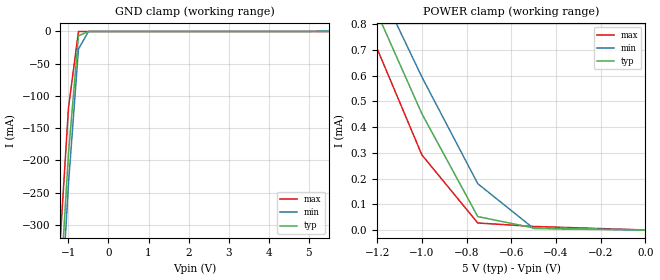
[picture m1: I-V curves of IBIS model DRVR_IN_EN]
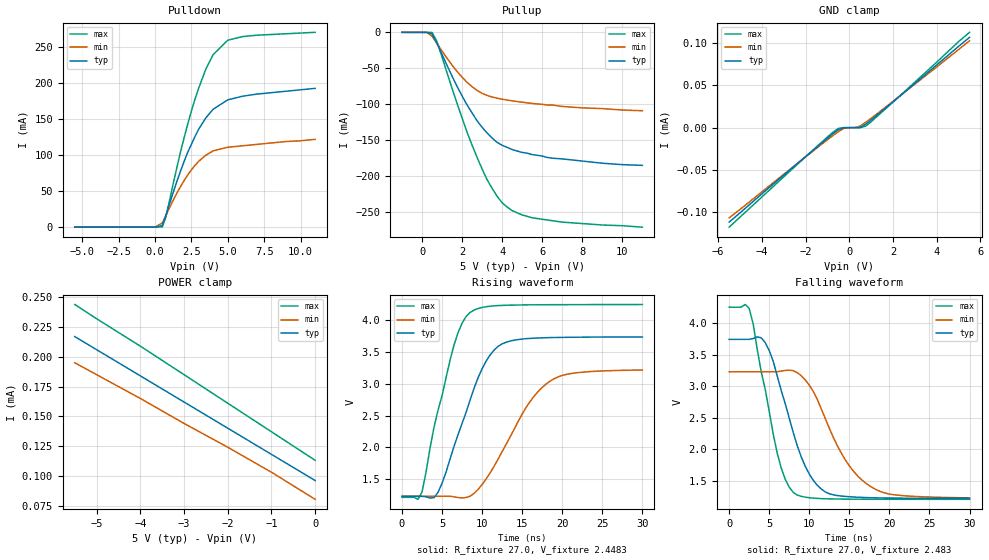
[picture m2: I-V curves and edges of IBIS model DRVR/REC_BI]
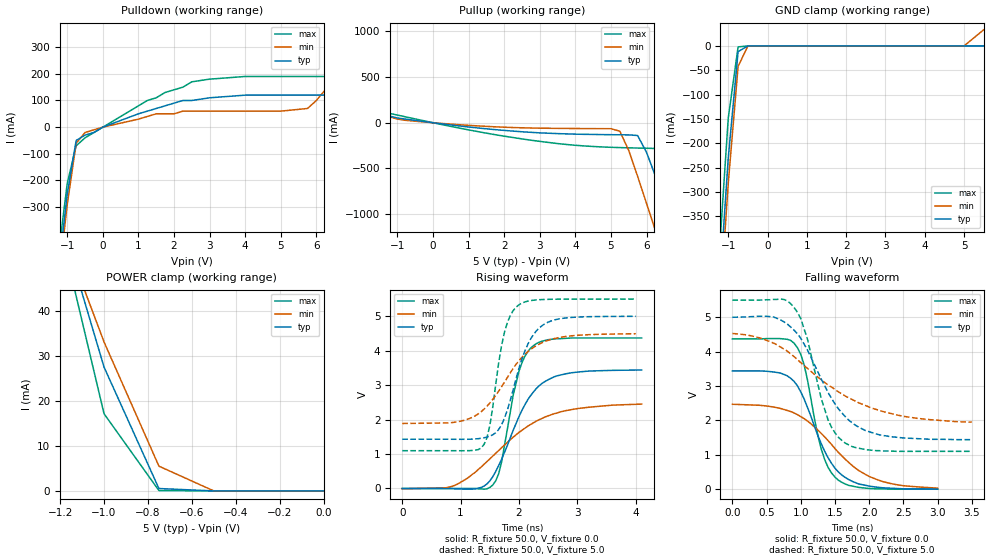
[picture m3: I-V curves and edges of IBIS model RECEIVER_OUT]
|   Texas Instruments Incorporated
|   Data Transmissions Products
|   IBIS Model for SN65HVD20
|   8D SOIC Package
[IBIS Ver]   3.2
[Comment char]   |_char
[File name]   sllc134a.ibs
[File Rev]   1.0
[Date]   9Dec02
[Source]   File originated at Texas Instruments Incorporated.
   Data Transmission Products Group.
[Notes]
[Disclaimer]
(C) Copyright Texas Instruments Incorporated 2002
   All rights reserved
  Texas Instruments Incorporated hereby grants the user of this IBIS
model a non-exclusive, nontransferable license to use this IBIS model
under the following terms.  Before using this IBIS model, the user
should read this license.  If the user does not accept these terms,
the IBIS model should be returned to Texas Instruments within 30 days.
  The user is granted this license only to use the IBIS model and
is not granted rights to sell, load, rent, lease or license the IBIS
model in whole or in part, or in modified form to anyone other than
user.  User may modify the IBIS model to suit its specific applications
but rights to derivative works and such modifications shall belong to
Texas Instruments.
  This IBIS model is provided on an "AS IS" basis and Texas Instruments
makes absolutely no warranty with respect to the information contained
herein.  TEXAS INSTRUMENTS DISCLAIMS AND CUSTOMER WAIVES ALL WARRANTIES,
EXPRESS OR IMPLIED, INCLUDING WARRANTIES OF MERCHANTABILITY OR FITNESS
FOR A PARTICULAR PURPOSE. The entire risk as to quality and performance
is with the Customer. ACCORDINGLY, IN NO EVENT SHALL THE COMPANY BE LIABLE
FOR ANY DAMAGES, WHETHER IN CONTRACT OR TORT,INCLUDING ANY LOST PROFITS
OR OTHER INCIDENTAL, CONSEQUENTIAL, EXEMPLARY, OR PUNITIVE DAMAGES ARISING
OUT OF THE USE OR APPLICATION OF THE IBIS model provided in this package.
Further, Texas Instruments reserves the right to discontinue or make changes
without notice to any product herein to improve reliability, function, or
design. Texas Instruments does not convey any license under patent rights
or any other intellectual property rights, including those of third parties.
Contact Texas Instruments at ATTN:DATA TRANSMISSIONS
[Copyright]   Copyright 2002, Texas Instruments, All Rights Reserved
[Component]   HVD20D
[Manufacturer]  Texas Instruments Incorporated
[Package]
|   typ   min   max
R_pkg   0.055   0.034   0.067
L_pkg   1.795nH   1.699nH   1.914nH
C_pkg   0.299pF   0.278pF   0.311pF
[Pin]   signal_name   model_name   R_pin   L_pin   C_pin
1   R   RECEIVER_OUT   0.067   1.914n   0.278p
2   RE   DRVR_IN_EN   0.062   1.816n   0.301p
3   DE   DRVR_IN_EN   0.053   1.699n   0.298p
4   D   DRVR_IN_EN   0.067   1.907n   0.278p
5   GND   GND   0.034   1.704n   0.311p
6   A   DRVR/REC_BI   0.061   1.808n   0.310p
7   B   DRVR/REC_BI   0.062   1.817n   0.302p
8   VCC   POWER   0.034   1.716n   0.311p
[Diff_pin]   inv_pin   vdiff   tdelay_typ   tdelay_min   tdelay_max
| The 'A' pin is Diff_pin and the 'B' pin is the inv_pin
6   7   0.200   0 0 0
| Models and submodels in the file (3): DRVR_IN_EN (Input), DRVR/REC_BI (I/O), RECEIVER_OUT (3-state)
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|   Driver Input / Receiver Enable Model
[Model]   DRVR_IN_EN
Model_type   Input
|Signals   D,DE,RE
Vinh = 2.0
Vinl = 0.8
|   typ   min   max
C_comp   1.0pF   NA   NA
|   typ   min   max
[Temperature Range]   25.0   -40   125
[Voltage range]   5.0V   4.5V   5.5V
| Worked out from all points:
|   GND clamp passes 1 mA (typ) near -0.54 V on its own axis
|   POWER clamp passes 1 mA (typ) near -1.28 V on its own axis
[GND_clamp]
|   Voltage   I(typ)   I(min)   I(max)
-5.5V     -4.7A      -4.83A     -4.52A
-2V       -1.22A     -1.29A     -1.12A
-1V       -190mA     -237mA     -119mA
-750mV    -6.83mA    -27.3mA    -170uA
-500mV    -28.3uA    -38.2uA    -58.3uA
5.5V      8.09uA     595uA      14.3pA
[Power_clamp]
| Note that the[POWER_clamp]voltage table is referenced to Vcc
| and is calculated using Vtable=Vcc - Vmeasured.
|   Voltage   I(typ)   I(min)   I(max)
-5.5V     9.83mA     9.25mA     10.5mA
-1.25V    941uA      1.05mA     808uA
-1V       452uA      595uA      292uA
-750mV    52uA       180uA      27.1uA
-500mV    8.09uA     5.88uA     13.7uA
0V        0A         0A         0A
|   Driver Output / Receiver Input Model
[Model]   DRVR/REC_BI
Model_type   I/O
| Signals   A,B
Vinl = 0.9V
Vinh = 2.8V
Vmeas = 1.7V   |Reference voltage for timing measurements
Cref = 50pF   |Timing specification test load capacitance value
Rref = 54   |Note: 54 Ohm load; single-ended configuration
|   Timing specification test load voltage
| variable   typ   min   max
C_comp   1.0pF   NA   NA
|   typ   min   max
[Temperature Range]   25.0   -40   85
[Voltage range]   5.0V   4.5V   5.5V
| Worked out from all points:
|   slope of the pulldown table from 0 to 0.75 V, typ, clamps not added: 47 ohm
|   slope of the pullup table from 0 to 0.75 V, typ, clamps not added: 49 ohm
|   rising waveform, R_fixture 27.0, V_fixture 2.4483: 20-80 % time 4.2ns typ, 5.45ns min, 3.29ns max; typ from 1.23 V to 3.74 V
|   falling waveform, R_fixture 27.0, V_fixture 2.483: 20-80 % time 3.68ns typ, 4.83ns min, 2.83ns max; typ from 3.74 V to 1.23 V
[Pulldown]
|   Voltage   I(typ)   I(min)   I(max)
-5.5V     -190uA     -172uA     -211uA
0V        -63.6uA    -53.6uA    -74.2uA
500mV     1.91mA     5.45mA     -1.94uA
750mV     15.9mA     15.9mA     13.6mA
1.75V     77.4mA     56.1mA     104mA
2.5V      115mA      79.5mA     161mA
3V        136mA      91.4mA     193mA
3.5V      152mA      100mA      220mA
4V        164mA      106mA      240mA
5V        177mA      111mA      260mA
6V        182mA      113mA      265mA
11V       193mA      122mA      271mA
[Pullup]
|   Voltage   I(typ)   I(min)   I(max)
| Note that the[Pullup]voltage table is referenced to Vcc
| and is calculated using Vtable=Vcc - Vmeasured.
-1V       132uA      115uA      155uA
250mV     89.9uA     -14.8uA    110uA
500mV     -1.84mA    -5.33mA    40.4uA
750mV     -15.2mA    -15.5mA    -12.7mA
1.75V     -75mA      -54.3mA    -98.8mA
2.25V     -101mA     -69.4mA    -139mA
2.75V     -123mA     -80.7mA    -174mA
3.5V      -147mA     -89.9mA    -217mA
4V        -157mA     -92.9mA    -237mA
4.25V     -160mA     -94.1mA    -243mA
5.5V      -170mA     -98.8mA    -258mA
11V       -185mA     -109mA     -271mA
[GND_clamp]
|   Voltage   I(typ)   I(min)   I(max)
| Outputs in High Impedance (off)
-5.5V     -112uA     -107uA     -118uA
-750mV    -7.21uA    -9.38uA    -5.43uA
-500mV    -2.33uA    -4.65uA    -907nA
-250mV    -20.5nA    -811nA     -9.78nA
250mV     -3.17nA    23.5nA     -3.43nA
500mV     217nA      1.95uA     -2.68nA
750mV     4.05uA     6.33uA     1.76uA
2V        30.6uA     31.2uA     30.3uA
5V        96.4uA     92.6uA     102uA
5.5V      107uA      103uA      113uA
[POWER_clamp]
|   Voltage   I(typ)   I(min)   I(max)
| Note that the [POWER_clamp] voltage table is referenced to Vcc
| and is calculated using Vtable = Vcc - Vmeasured.
| Outputs in Tri-state.
-5.5V     217uA      195uA      244uA
-5V       206uA      185uA      232uA
-4V       184uA      165uA      209uA
-3V       162uA      144uA      185uA
-2V       140uA      124uA      161uA
-1V       118uA      103uA      137uA
0V        96uA       80.2uA     113uA
[Ramp]
|   typ   min   max
dV/dt_r   1.51V/4.21ns   1.19V/5.45ns   1.82V/3.29ns
dV/dt_f   1.51V/3.67ns   1.20V/4.83ns   1.82V/3.43ns
R_load = 27ohm | Note: The measurement is on a single-ended configuration
|   with 54ohm line-to-line.
[Rising Waveform]
R_fixture = 27.0
V_fixture = 2.4483
V_fixture_min = 2.227
V_fixture_max = 2.73
C_fixture = 0p
L_fixture = 0n
|   V(typ)   V(min)   V(max)
0s        1.227V     1.228V     1.211V
2.5ns     1.227V     1.228V     1.296V
4.5ns     1.29V      1.228V     2.583V
7ns       2.199V     1.208V     3.805V
8.5ns     2.744V     1.229V     4.122V
10ns      3.237V     1.414V     4.202V
12ns      3.589V     1.815V     4.231V
15.5ns    3.71V      2.628V     4.242V
18ns      3.725V     2.996V     4.244V
30ns      3.737V     3.216V     4.248V
[Falling Waveform]
R_fixture = 27.0
V_fixture = 2.483
V_fixture_min = 2.227
V_fixture_max = 2.73
C_fixture = 0p
L_fixture = 0n
|   V(typ)   V(min)   V(max)
0s        3.74V      3.227V     4.249V
2.5ns     3.74V      3.227V     4.229V
5ns       3.563V     3.227V     2.601V
6.5ns     2.93V      3.239V     1.705V
8ns       2.265V     3.245V     1.322V
9.5ns     1.733V     3.098V     1.246V
11.5ns    1.374V     2.64V      1.223V
14.5ns    1.258V     1.834V     1.215V
17ns      1.24V      1.472V     1.213V
30ns      1.228V     1.235V     1.212V
|   Receiver Output Model
[Model]   RECEIVER_OUT
Model_type   3-state
| Signals   R
Vmeas = 2.2V   |Reference voltage for timing measurements
Cref = 15pF   |Timing specification test load capacitance value
Vref = 0   |Timing specification test load voltage; GND
| variable   typ   min   max
C_comp   1.0pF   NA   NA
|   typ   min   max
[Temperature Range]   25.0   -40   85
[Voltage range]   5.0V   4.5V   5.5V
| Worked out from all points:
|   slope of the pulldown table from 0 to 0.75 V, typ, clamps not added: 20 ohm
|   slope of the pullup table from 0 to 0.75 V, typ, clamps not added: 21 ohm
|   GND clamp passes 1 mA (typ) near -0.52 V on its own axis
|   POWER clamp passes 1 mA (typ) near -0.75 V on its own axis
|   rising waveform, R_fixture 50.0, V_fixture 0.0: 20-80 % time 566ps typ, 1.04ns min, 306ps max; typ from 0 V to 3.44 V
|   falling waveform, R_fixture 50.0, V_fixture 0.0: 20-80 % time 454ps typ, 770ps min, 285ps max; typ from 3.44 V to 0 V
|   rising waveform, R_fixture 50.0, V_fixture 5.0: 20-80 % time 409ps typ, 689ps min, 252ps max; typ from 1.43 V to 5 V
|   falling waveform, R_fixture 50.0, V_fixture 5.0: 20-80 % time 602ps typ, 1.1ns min, 351ps max; typ from 5 V to 1.44 V
[Pulldown]
|   Voltage   I(typ)   I(min)   I(max)
-5.5V     -5.53A     -5.49A     -5.57A
-1.25V    -540mA     -580mA     -480mA
-1V       -250mA     -290mA     -210mA
-750mV    -50mA      -60mA      -70mA
-500mV    -30mA      -20mA      -40mA
1.25V     60mA       40mA       100mA
2.5V      100mA      60mA       170mA
5.75V     120mA      70mA       190mA
6.5V      130mA      170mA      190mA
7.25V     250mA      270mA      200mA
8V        380mA      380mA      360mA
11V       920mA      800mA      1.05A
[Pullup]
|   Voltage   I(typ)   I(min)   I(max)
| Note that the[Pullup]voltage table is referenced to Vcc
| and is calculated using Vtable=Vcc - Vmeasured.
-5.5V     831mA      660mA      1.05A
-1.5V     116mA      101mA      135mA
-750mV    38.6mA     25.2mA     62.6mA
1.5V      -66.6mA    -39.9mA    -114mA
5.25V     -132mA     -93mA      -272mA
5.75V     -140mA     -586mA     -277mA
6V        -324mA     -882mA     -279mA
6.25V     -583mA     -1.18A     -282mA
6.5V      -849mA     -1.47A     -402mA
7V        -1.44A     -2.06A     -909mA
8V        -2.62A     -3.21A     -1.99A
11V       -6.03A     -6.64A     -5.58A
[GND_clamp]
|   Voltage   I(typ)   I(min)   I(max)
| Outputs in High Impedance (off)
-5.5V     -5.53A     -5.49A     -5.57A
-1.25V    -531mA     -579mA     -452mA
-1V       -230mA     -282mA     -148mA
-750mV    -11.8mA    -42mA      -2.02mA
-500mV    -7.54uA    -155uA     -41.3uA
5V        0A         5.88uA     -7.45nA
5.5V      22.4nA     33.2mA     -7.45nA
[POWER_clamp]
|   Voltage   I(typ)   I(min)   I(max)
| Note that the [POWER_clamp] voltage table is referenced to Vcc
| and is calculated using Vtable = Vcc - Vmeasured.
| Outputs in Tri-state.
-5.5V     845mA      659mA      1.05A
-1.25V    68.8mA     65.7mA     68.8mA
-1V       27.6mA     33.2mA     17.2mA
-750mV    537uA      5.52mA     88.4uA
-500mV    22.4nA     5.88uA     0A
0V        0A         0A         -7.45nA
[Ramp]
|   typ   min   max
dV/dt_r   2.06V/563ps   1.47V/1038ps   2.62V/306ps
dV/dt_f   2.14V/599ps   1.55V/1103ps   2.64V/346ps
R_load = 50
[Rising Waveform]
R_fixture = 50.0
V_fixture = 0.0
C_fixture = 0p
L_fixture = 0n
|   V(typ)   V(min)   V(max)
0s        0V         -10mV      0V
900ps     -10mV      90mV       0V
1.35ns    30mV       620mV      -10mV
1.55ns    340mV      940mV      100mV
1.7ns     840mV      1.18V      760mV
1.9ns     1.69V      1.49V      2.71V
2ns       2.09V      1.63V      3.41V
2.3ns     2.91V      1.96V      4.21V
2.9ns     3.36V      2.29V      4.37V
4.1ns     3.44V      2.45V      4.37V
[Falling Waveform]
R_fixture = 50.0
V_fixture = 0.0
C_fixture = 0p
L_fixture = 0n
|   V(typ)   V(min)   V(max)
0s        3.44V      2.47V      4.37V
700ps     3.38V      2.35V      4.38V
950ps     3.01V      2.17V      4.12V
1.05ns    2.62V      2.05V      3.61V
1.3ns     1.32V      1.62V      1.16V
1.4ns     910mV      1.41V      630mV
1.55ns    500mV      1.07V      260mV
1.8ns     190mV      610mV      70mV
2.1ns     60mV       290mV      10mV
3ns       0V         30mV       0V
[Rising Waveform]
R_fixture = 50.0
V_fixture = 5.0
V_fixture_min = 4.5
V_fixture_max = 5.5
C_fixture = 0p
L_fixture = 0n
|   V(typ)   V(min)   V(max)
0s        1.43V      1.887V     1.097V
950ps     1.428V     1.938V     1.096V
1.4ns     1.472V     2.302V     1.276V
1.5ns     1.519V     2.481V     1.827V
1.65ns    1.709V     2.822V     3.631V
1.75ns    2.037V     3.084V     4.53V
2ns       3.497V     3.713V     5.336V
2.2ns     4.345V     4.039V     5.456V
2.5ns     4.831V     4.303V     5.492V
4ns       4.999V     4.493V     5.5V
[Falling Waveform]
R_fixture = 50.0
V_fixture = 5.0
V_fixture_min = 4.5
V_fixture_max = 5.5
C_fixture = 0p
L_fixture = 0n
|   V(typ)   V(min)   V(max)
0s        5V         4.53V      5.5V
600ps     5.01V      4.25V      5.52V
900ps     4.63V      3.86V      5.29V
1ns       4.39V      3.68V      4.96V
1.1ns     4.04V      3.51V      4.35V
1.3ns     3.2V       3.18V      2.63V
1.4ns     2.81V      3.03V      2.01V
1.65ns    2.11V      2.71V      1.34V
2.2ns     1.56V      2.26V      1.11V
3.5ns     1.44V      1.95V      1.1V
